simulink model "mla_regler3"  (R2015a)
settings: Solver=ode5  StartTime=0.0  StopTime=10  FixedStep=0.0001  RelTol=1e-3
PreLoadFcn:
  | MLA_Sensor1 = load('mla_sensor1.dat');
libraries: libmla x1, simulink_need_slupdate x1, slrtlib x1

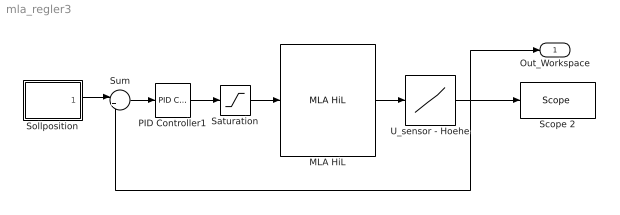
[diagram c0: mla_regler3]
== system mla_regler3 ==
  MLA HiL : libmla/MLA HiL  SystemSampleTime=-1
  PID Controller1 : simulink_need_slupdate/PID Controller  P=9000  I=2000  D=100
  Saturation : Saturate  UpperLimit=3  LowerLimit=-3
  Scope 2 : slrtlib/Displays and Logging/Scope   scopeno=1  scopetype=Target  autostart=on  viewmode=Graphical sliding  formatstr='%15.6f'  grid=on  ylimits=[0 0.132]  nosamples=1000  noprepostsamples=0  interleave=10  triggermode=FreeRun  triggersignal=1  trigsignalfromport=off  triggerlevel=0.0  triggerslope=Either  triggerscope=1  triggersample=0  filename=data.dat  mode=Lazy  writesize=512  autorestart=off  dynamicfilemode=off  maxwritefilesize=512*1024^2
  Sollposition : Subsystem
  Sum : Sum  Inputs=|+-
  U_sensor - Hoehe : Lookup  InputValues=MLA_Sensor1(:,1)  Table=MLA_Sensor1(:,2)
  Out_Workspace : Outport
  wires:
  U_sensor - Hoehe/1 -> Out_Workspace/1, Scope 2/1, Sum/2
  Saturation/1 -> MLA HiL/1
  MLA HiL/1 -> U_sensor - Hoehe/1
  PID Controller1/1 -> Saturation/1
  Sum/1 -> PID Controller1/1
  Sollposition/1(Sollwert) -> Sum/1

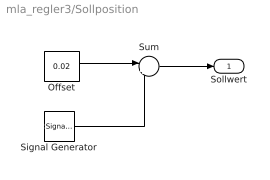
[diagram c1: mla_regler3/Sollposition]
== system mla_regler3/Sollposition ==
  Offset : Constant  Value=0.02
  Signal Generator : SignalGenerator  Amplitude=0.01  Frequency=0.5
  Sum : Sum  Inputs=|++
  Sollwert : Outport
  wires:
  Signal Generator/1 -> Sum/2
  Sum/1 -> Sollwert/1
  Offset/1 -> Sum/1
